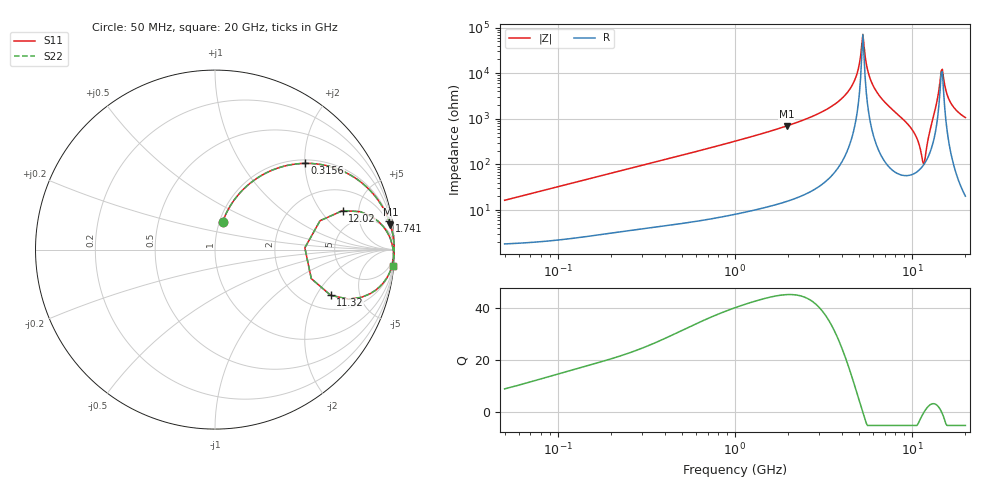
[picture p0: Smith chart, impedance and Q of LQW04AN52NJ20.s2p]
!Murata Part Number: LQW04AN52NJ20
!These Parameters are Measured in Series Mode Connection
!  o--[Z]--o
!Port1  Port2
!  o-------o
!Freq. Start=50[MHz] Stop=20[GHz], 401[Steps]
# Hz S RI R 50
!Freq.(Hz) S11(Real) S11(Imag) S21(Real) S21(Imag) S12(Real) S12(Imag) S22(Real) S22(Imag)
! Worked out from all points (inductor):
!   401 points, 50 MHz to 20 GHz, reference 50 ohm
!   read as one part in series: L = 51.8 nH near 51.52 MHz
!   highest Q = 45 at 1.962 GHz (marker M1), where L = 56.7 nH
!   self-resonance near 5.273 GHz
!   S11 on the Smith chart (normalised r, x): 50 MHz: 1.04, +0.33; 315.6 MHz: 1.08, +2.01; 1.741 GHz: 1, +12; 11.32 GHz: 2.72, -2.66; 12.02 GHz: 3.42, +3.32; 20 GHz: 1, -21
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5e7  0.0424 0.1534  0.9576 -0.1534  0.9576 -0.1534  0.0424 0.1534
1.364002e8  0.1769 0.3537  0.8231 -0.3537  0.8231 -0.3537  0.1769 0.3537
3.155756e8  0.5031 0.4805  0.4969 -0.4805  0.4969 -0.4805  0.5031 0.4805
3.721004e8  0.581 0.4754  0.419 -0.4754  0.419 -0.4754  0.581 0.4754
1e9  0.907 0.2782  0.093 -0.2782  0.093 -0.2782  0.907 0.2782
1.740566e9  0.9697 0.1605  0.0303 -0.1605  0.0303 -0.1605  0.9697 0.1605
1.962148e9  0.977 0.1393  0.023 -0.1393  0.023 -0.1393  0.977 0.1393
2.728004e9  0.9902 0.0876  0.00982 -0.0876  0.00982 -0.0876  0.9902 0.0876
4.34015e9  0.998 0.0255  0.00205 -0.0255  0.00205 -0.0255  0.998 0.0255
4.81993e9  0.9985 0.0119  0.00152 -0.0119  0.00152 -0.0119  0.9985 0.0119
5.273168e9  0.9986 3.41e-05  0.00141 -3.41e-05  0.00141 -3.41e-05  0.9986 3.41e-05
5.944466e9  0.9982 -0.0166  0.00184 0.0166  0.00184 0.0166  0.9982 -0.0166
7.442007e9  0.9945 -0.0538  0.00546 0.0538  0.00546 0.0538  0.9945 -0.0538
1.019291e10  0.9447 -0.1762  0.0553 0.1762  0.0553 0.1762  0.9447 -0.1762
1.131968e10  0.6443 -0.2545  0.3557 0.2545  0.3557 0.2545  0.6443 -0.2545
1.201863e10  0.711 0.2173  0.289 -0.2173  0.289 -0.2173  0.711 0.2173
1.276073e10  0.9383 0.1276  0.0617 -0.1276  0.0617 -0.1276  0.9383 0.1276
1.375312e10  0.9837 0.0411  0.0163 -0.0411  0.0163 -0.0411  0.9837 0.0411
1.438523e10  0.9906 0.0115  0.0094 -0.0115  0.0094 -0.0115  0.9906 0.0115
1.482269e10  0.9928 -0.00374  0.00723 0.00374  0.00723 0.00374  0.9928 -0.00374
1.670968e10  0.9943 -0.0473  0.00569 0.0473  0.00569 0.0473  0.9943 -0.0473
2e10  0.9895 -0.0928  0.0105 0.0928  0.0105 0.0928  0.9895 -0.0928
